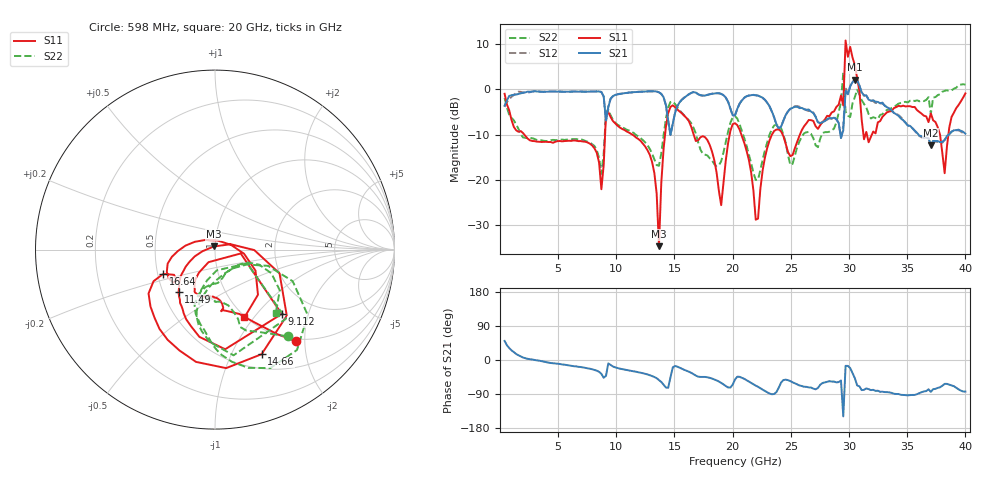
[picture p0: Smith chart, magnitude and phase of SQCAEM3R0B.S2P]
! Network Analyzer HP8722ES.07.66: Jul 25, 2000 Serial No. US39175408
! 26 Oct 2004  13:32:47
! Frequency  S11  S21  S12  S22
# HZ  S  DB R  50
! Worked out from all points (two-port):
!   201 points, 400 MHz to 40 GHz, reference 50 ohm
!   highest |S21| = 2.06 dB at 30.5 GHz (marker M1); lowest = -12.4 dB at 37.03 GHz (marker M2)
!   |S21| within 3 dB of the highest: 1.759 GHz to 8.778 GHz (7.018 GHz wide, 133 % of centre); 10.58 GHz to 13.81 GHz (3.233 GHz wide, 26.5 % of centre)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
!   lowest |S11| = -34.6 dB at 13.67 GHz (marker M3), VSWR 1.04, Z = 49.3 + j1.71 ohm
!   |S11| at or under -10 dB: 2.088 GHz to 9.036 GHz (6.948 GHz wide, 125 % of centre); 11.36 GHz to 14.19 GHz (2.827 GHz wide, 22.1 % of centre); 16.65 GHz to 19.74 GHz (3.098 GHz wide, 17 % of centre)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
!   |S22| runs from -20.0 to 3.7 dB; largest |S21 - S12| = 0.27
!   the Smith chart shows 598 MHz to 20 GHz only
!   S11 on the Smith chart (normalised r, x): 598 MHz: 0.96, -1.81; 9.112 GHz: 1.40, -1.37; 11.49 GHz: 0.60, -0.31; 14.66 GHz: 0.67, -1.31; 16.64 GHz: 0.53, -0.16; 20 GHz: 0.99, -0.90
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4e8  -1.02 -41.1  -3.64 50.3  -3.91 55.8  -1.96 -32.8
5.98e8  -3.36 -48.6  -2.47 38.9  -2.86 40.2  -4.02 -50.1
7.132e9  -11.53 -113.5  -0.54 -19.6  -0.56 -19.8  -11.21 -106.4
9.112e9  -5.74 -44.0  -6.89 -42.0  -7.17 -40.8  -5.16 -44.2
1.1488e10  -10.19 -131.0  -0.65 -29.7  -0.69 -29.6  -9.63 -106.3
1.3666e10  -34.61 110.9  -0.70 -52.9  -0.69 -52.6  -16.88 -47.1
1.4656e10  -3.90 -66.0  -10.06 -45.4  -10.13 -43.8  -2.83 -50.8
1.6636e10  -9.92 -154.8  -0.66 -37.6  -0.62 -37.1  -8.53 -106.7
2.0002e10  -7.71 -66.5  -5.77 -65.1  -5.84 -64.2  -6.21 -46.2
2.02e10  -7.50 -86.4  -5.81 -51.2  -5.68 -50.3  -5.94 -60.9
2.1982e10  -28.77 -109.9  -1.34 -67.6  -1.34 -67.2  -20.01 -60.1
2.6932e10  -7.01 -60.0  -5.26 -75.6  -5.18 -75.1  -10.81 -22.1
2.9506e10  -3.59 8.4  -9.06 -148.8  -8.03 -124.3  3.70 34.5
2.9704e10  10.74 -4.0  -0.40 -15.4  0.30 -0.7  -4.95 -49.5
2.9902e10  7.14 -59.1  -1.10 -15.6  -1.13 -15.7  -5.83 14.1
3.01e10  9.33 -74.9  0.57 -21.2  0.72 -21.0  -6.14 20.8
3.0496e10  5.37 -98.2  2.06 -47.7  1.96 -46.7  -1.77 -2.2
3.0694e10  2.41 54.3  2.06 -66.9  2.01 -66.1  -0.11 161.8
3.1486e10  -9.42 -92.3  -1.39 -75.0  -1.41 -75.3  -4.01 -33.6
3.3466e10  -4.92 -36.2  -4.24 -85.5  -4.46 -84.6  -4.49 -3.5
3.703e10  -5.33 -70.9  -12.39 -84.2  -12.46 -83.3  -5.50 21.9
4e10  -0.93 -34.5  -9.80 -83.5  -10.09 -83.2  1.01 -0.5
